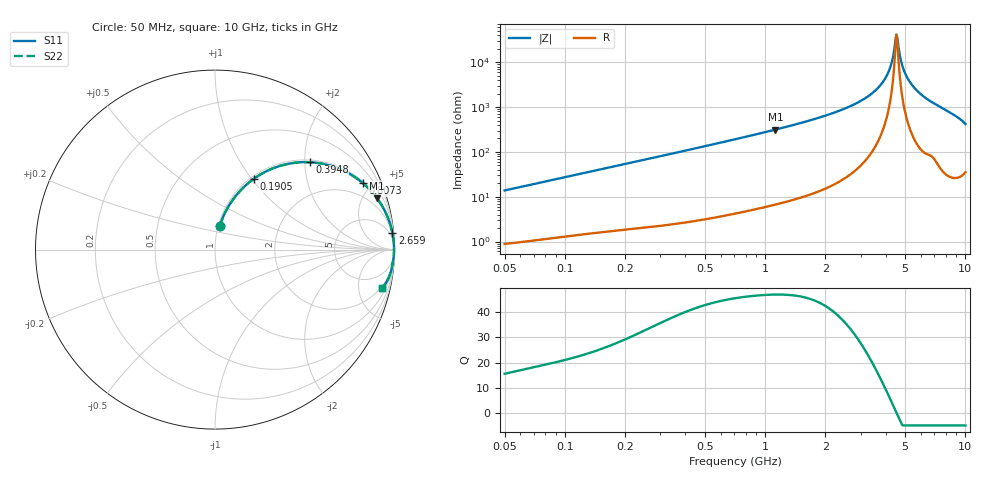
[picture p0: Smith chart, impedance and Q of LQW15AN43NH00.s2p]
!Murata Part Number: LQW15AN43NH00
!These Parameters are Measured in Series Mode Connection
!  o--[Z]--o
!Port1  Port2
!  o-------o
!Freq. Start=50[MHz] Stop=10[GHz], 401[Steps]
# Hz S RI R 50
!Freq.(Hz)	S 11(Real)	S 11(Imag)	S 21(Real)	S 21(Imag)	S 12(Real)	S 12(Imag)	S 22(Real)	S 22(Imag)
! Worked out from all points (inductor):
!   401 points, 50 MHz to 10 GHz, reference 50 ohm
!   read as one part in series: L = 43.6 nH near 51.34 MHz
!   highest Q = 47.1 at 1.124 GHz (marker M1), where L = 44.5 nH
!   self-resonance near 4.517 GHz
!   S11 on the Smith chart (normalised r, x): 50 MHz: 1.02, +0.28; 190.5 MHz: 1.04, +1.02; 394.8 MHz: 1.05, +2.11; 807.3 MHz: 1.09, +4.39; 2.659 GHz: 2, +21; 10 GHz: 1.71, -8.38
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5e7  0.0269 0.1328  0.9731 -0.1328  0.9731 -0.1328  0.0269 0.1328
1.214486e8  0.1077 0.2889  0.8923 -0.2889  0.8923 -0.2889  0.1077 0.2889
1.905373e8  0.2154 0.394  0.7846 -0.394  0.7846 -0.394  0.2154 0.394
2.949953e8  0.3867 0.4731  0.6133 -0.4731  0.6133 -0.4731  0.3867 0.4731
3.947951e8  0.5265 0.4869  0.4735 -0.4869  0.4735 -0.4869  0.5265 0.4869
7.071068e8  0.7802 0.4033  0.2198 -0.4033  0.2198 -0.4033  0.7802 0.4033
8.07255e8  0.823 0.371  0.177 -0.371  0.177 -0.371  0.823 0.371
1.124152e9  0.9031 0.2855  0.0969 -0.2855  0.0969 -0.2855  0.9031 0.2855
1.717543e9  0.9609 0.183  0.0391 -0.183  0.0391 -0.183  0.9609 0.183
2.659148e9  0.9882 0.0941  0.0118 -0.0941  0.0118 -0.0941  0.9882 0.0941
3.558764e9  0.9958 0.0419  0.00417 -0.0419  0.00417 -0.0419  0.9958 0.0419
3.904516e9  0.997 0.0259  0.00301 -0.0259  0.00301 -0.0259  0.997 0.0259
4.171863e9  0.9975 0.0144  0.00252 -0.0144  0.00252 -0.0144  0.9975 0.0144
4.283859e9  0.9976 0.00983  0.0024 -0.00983  0.0024 -0.00983  0.9976 0.00983
4.457516e9  0.9977 0.00292  0.00231 -0.00292  0.00231 -0.00292  0.9977 0.00292
4.577181e9  0.9977 -0.0017  0.00231 0.0017  0.00231 0.0017  0.9977 -0.0017
4.826234e9  0.9975 -0.011  0.00246 0.011  0.00246 0.011  0.9975 -0.011
4.955797e9  0.9974 -0.0157  0.00261 0.0157  0.00261 0.0157  0.9974 -0.0157
5.225452e9  0.9969 -0.0253  0.00308 0.0253  0.00308 0.0253  0.9969 -0.0253
5.583245e9  0.996 -0.0375  0.00402 0.0375  0.00402 0.0375  0.996 -0.0375
6.458996e9  0.9917 -0.0659  0.00832 0.0659  0.00832 0.0659  0.9917 -0.0659
1e10  0.9301 -0.2162  0.0699 0.2162  0.0699 0.2162  0.9301 -0.2162
